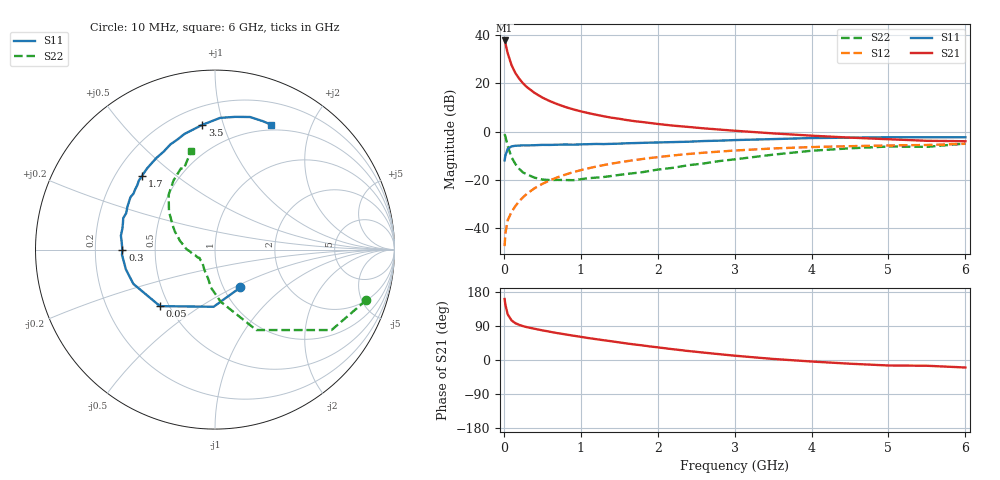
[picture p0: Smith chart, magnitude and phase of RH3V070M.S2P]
! SIEMENS Small Signal Semiconductors
! BFR106
! Si NPN RF Bipolar Junction Transistor in SOT23
! VCE = 3 V  IC = 70 mA
! Common Emitter S-Parameters:  August  1996
# GHz  S  MA  R  50
!  f  S11  S21  S12  S22
! GHz  MAG  ANG  MAG  ANG  MAG  ANG  MAG  ANG
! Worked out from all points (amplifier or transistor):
!   36 points, 10 MHz to 6 GHz, reference 50 ohm
!   highest |S21| = 37.8 dB at 10 MHz (marker M1)
!   |S21| within 3 dB of that: start of sweep to 33.26 MHz
!   unconditionally stable (mu >= 1): 198.4 MHz to 2.515 GHz; 5.481 GHz to end of sweep
!   at 250 MHz: K = 1.04, MAG = 22.4 dB, |S12| = -27.3 dB
!   at 1.4 GHz: K = 1.07, MAG = 8.0 dB, |S12| = -13.3 dB
!   at 6 GHz: K = 1.00, MAG = 0.4 dB, |S12| = -5.1 dB
!   S11 on the Smith chart (normalised r, x): 10 MHz: 1.20, -0.54; 50 MHz: 0.45, -0.35; 300 MHz: 0.32, -0.00; 1.7 GHz: 0.31, +0.38; 3.5 GHz: 0.31, +0.85; 6 GHz: 0.44, +1.46
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0.01  0.2538 -56.1  77.7 161.0  0.0042 77.7  0.8893 -18.4
0.02  0.3186 -91.4  67.72 146.0  0.0077 67.2  0.7892 -34.6
0.05  0.4394 -134.2  42.3 120.5  0.0145 61.3  0.5038 -62.8
0.1  0.4933 -157.2  23.99 104.5  0.0215 64.2  0.2931 -83.6
0.15  0.5086 -167.5  16.39 97.1  0.0285 67.1  0.2128 -96.1
0.2  0.5124 -172.5  12.51 92.7  0.0361 70.1  0.1682 -102.8
0.25  0.5191 -176.8  9.998 89.3  0.0434 71.1  0.1419 -110.8
0.3  0.516 -179.7  8.376 86.7  0.0514 72.5  0.1296 -116.6
0.4  0.5219 175.2  6.342 82.4  0.0669 73.2  0.1107 -126.5
0.5  0.53 171.6  5.086 78.3  0.0821 72.6  0.1013 -133.4
0.6  0.5291 167.3  4.269 74.5  0.0979 71.8  0.0987 -138.2
0.7  0.5342 163.7  3.684 70.8  0.1131 70.9  0.0995 -143.3
0.8  0.5405 161.1  3.238 67.6  0.1282 69.4  0.0989 -148.6
1.1  0.5481 151.1  2.416 57.9  0.1732 65.4  0.108 -157.3
1.4  0.557 143.0  1.942 49.4  0.2162 60.5  0.12 -166.0
1.7  0.5775 134.9  1.645 40.9  0.2569 55.8  0.1379 -175.2
2.2  0.606 122.6  1.33 28.4  0.3203 47.7  0.1775 171.9
2.8  0.6482 108.8  1.103 15.4  0.3848 37.9  0.2445 155.9
3.5  0.6987 95.8  0.918 2.8  0.4468 27.1  0.3323 140.5
4.5  0.748 81.4  0.75 -9.8  0.4982 12.7  0.4496 120.9
5.5  0.7636 69.5  0.644 -15.2  0.5276 3.6  0.4828 111.1
6  0.763 65.8  0.631 -19.8  0.5579 -3.3  0.564 103.7
